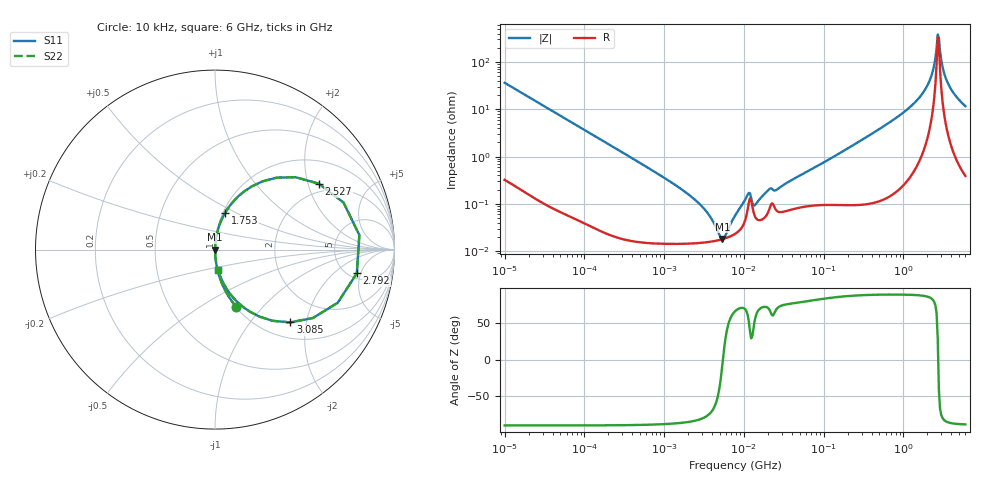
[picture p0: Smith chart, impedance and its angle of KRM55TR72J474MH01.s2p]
!Murata Part Number: KRM55TR72J474MH01
!These Parameters are Measured in Series Mode Connection
!Data Generated on Jan 08, 2026
!  o--ll--o
!Port1  Port2
!  o------o
!Operation Temp=25[degC], DC Bias Voltage=0[V]
!Freq. Start=10[kHz] Stop=6[GHz] 401[Steps]
# Hz S RI R 50
!Freq.(Hz) S11(Real) S11(Imag) S21(Real) S21(Imag) S12(Real) S12(Imag) S22(Real) S22(Imag)
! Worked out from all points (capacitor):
!   401 points, 10 kHz to 6 GHz, reference 50 ohm
!   read as one part in series: C = 437 nF near 10.69 kHz
!   lowest |Z| = 18.1 mohm at 5.373 MHz (marker M1)
!   series resonance near 5.462 MHz, so ESL is about 1.9 nH
!   S11 on the Smith chart (normalised r, x): 10 kHz: 1.01, -0.73; 1.753 GHz: 1.02, +0.44; 2.527 GHz: 1.70, +2.36; 2.792 GHz: 5.85, -4.29; 3.085 GHz: 1.31, -1.62; 6 GHz: 1.01, -0.23
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10000  0.1191 -0.3195  0.8809 0.3195  0.8809 0.3195  0.1191 -0.3195
28042  0.0178 -0.128  0.9822 0.128  0.9822 0.128  0.0178 -0.128
92862  0.00198 -0.0395  0.998 0.0395  0.998 0.0395  0.00198 -0.0395
862344  0.000162 -0.00418  0.9998 0.00418  0.9998 0.00418  0.000162 -0.00418
2855711  0.000151 -0.000946  0.9998 0.000946  0.9998 0.000946  0.000151 -0.000946
5372501  0.00018 -2.27e-05  0.9998 2.27e-05  0.9998 2.27e-05  0.00018 -2.27e-05
7745967  0.000233 0.000514  0.9998 -0.000514  0.9998 -0.000514  0.000233 0.000514
1.116798e7  0.000771 0.00137  0.9992 -0.00137  0.9992 -0.00137  0.000771 0.00137
1.409589e7  0.000508 0.000846  0.9995 -0.000846  0.9995 -0.000846  0.000508 0.000846
2.101053e7  0.0008 0.00193  0.9992 -0.00193  0.9992 -0.00193  0.0008 0.00193
2.565129e7  0.00073 0.00185  0.9993 -0.00185  0.9993 -0.00185  0.00073 0.00185
7.193098e7  0.000947 0.00543  0.9991 -0.00543  0.9991 -0.00543  0.000947 0.00543
6.67969e8  0.00417 0.0523  0.9958 -0.0523  0.9958 -0.0523  0.00417 0.0523
1.752557e9  0.0564 0.205  0.9436 -0.205  0.9436 -0.205  0.0564 0.205
2.212024e9  0.2069 0.3532  0.7931 -0.3532  0.7931 -0.3532  0.2069 0.3532
2.364181e9  0.3428 0.4007  0.6572 -0.4007  0.6572 -0.4007  0.3428 0.4007
2.526803e9  0.5793 0.3671  0.4207 -0.3671  0.4207 -0.3671  0.5793 0.3671
2.791949e9  0.7903 -0.1315  0.2097 0.1315  0.2097 0.1315  0.7903 -0.1315
3.084918e9  0.4192 -0.4055  0.5808 0.4055  0.5808 0.4055  0.4192 -0.4055
3.40863e9  0.1952 -0.3464  0.8048 0.3464  0.8048 0.3464  0.1952 -0.3464
3.766309e9  0.1045 -0.271  0.8955 0.271  0.8955 0.271  0.1045 -0.271
6e9  0.0171 -0.1141  0.9829 0.1141  0.9829 0.1141  0.0171 -0.1141
